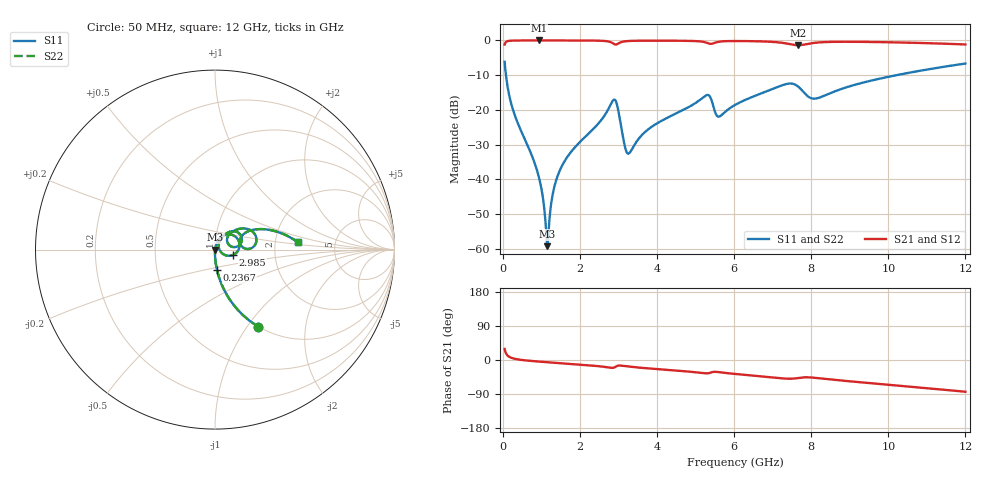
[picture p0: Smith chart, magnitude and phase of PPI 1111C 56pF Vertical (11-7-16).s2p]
# GHz S MA R 50
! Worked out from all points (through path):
!   1601 points, 50 MHz to 12 GHz, reference 50 ohm
!   highest |S21| = -0.01 dB at 938.8 MHz (marker M1); lowest = -1.4 dB at 7.661 GHz (marker M2)
!   group delay of S21, straight-line fit = 19.3 ps
!   lowest |S11| = -59.3 dB at 1.155 GHz (marker M3), VSWR 1.00, Z = 50.1 - j0.0227 ohm
!   |S11| at or under -10 dB: 84.54 MHz to 10.22 GHz (10.13 GHz wide, 197 % of centre)
!   |S22| runs from -59.3 to -6.2 dB; largest |S21 - S12| = 0
!   S11 on the Smith chart (normalised r, x): 50 MHz: 1.00, -1.13; 236.7 MHz: 1.00, -0.23; 2.985 GHz: 1.22, -0.07; 12 GHz: 2.70, +0.28
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0.05  0.492 -60.8  0.8703 29.2  0.8703 29.2  0.492 -60.8
0.2367188  0.114 -84.4  0.9929 5.3  0.9929 5.3  0.114 -84.4
0.9387813  0.01072 -89.0  0.9989 -4.2  0.9989 -4.2  0.01072 -89.0
1.028406  0.006133 -85.4  0.9989 -4.9  0.9989 -4.9  0.006133 -85.4
1.155375  0.001084 -12.1  0.9989 -5.9  0.9989 -5.9  0.001084 -12.1
1.192719  0.00188 48.1  0.9988 -6.2  0.9988 -6.2  0.00188 48.1
1.30475  0.006359 72.4  0.9987 -7.1  0.9987 -7.1  0.006359 72.4
1.439188  0.01172 75.8  0.9986 -8.0  0.9986 -8.0  0.01172 75.8
2.044156  0.03623 74.2  0.9971 -12.5  0.9971 -12.5  0.03623 74.2
2.85825  0.1357 30.9  0.9099 -20.7  0.9099 -20.7  0.1357 30.9
2.985219  0.106 -16.1  0.8938 -15.1  0.8938 -15.1  0.106 -16.1
3.164469  0.03042 -16.2  0.9694 -16.1  0.9694 -16.1  0.03042 -16.2
3.254094  0.02333 15.2  0.98 -17.3  0.98 -17.3  0.02333 15.2
4.038312  0.06545 60.8  0.9919 -24.2  0.9919 -24.2  0.06545 60.8
5.285594  0.1627 32.8  0.9275 -35.2  0.9275 -35.2  0.1627 32.8
5.591812  0.07968 25.4  0.9543 -31.9  0.9543 -31.9  0.07968 25.4
6.025  0.1175 46.9  0.9799 -36.8  0.9799 -36.8  0.1175 46.9
7.302156  0.231 26.1  0.9147 -48.9  0.9147 -48.9  0.231 26.1
7.660656  0.2168 4.6  0.8518 -47.5  0.8518 -47.5  0.2168 4.6
8.019156  0.1461 10.6  0.9124 -46.3  0.9124 -46.3  0.1461 10.6
10.01331  0.3 22.2  0.941 -65.4  0.941 -65.4  0.3 22.2
12  0.4646 4.9  0.8748 -83.8  0.8748 -83.8  0.4646 4.9
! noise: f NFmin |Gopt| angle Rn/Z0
0.05  0.0003756  0.8674  0.5859  0.0006088
1.372  0.003976  0.6895  7  0.002482
2.701  0.02314  0.8839  13.75  0.04262
4.031  0.01462  0.7492  20.26  0.01138
5.36  0.07012  0.925  26.87  0.1959
6.682  0.03075  0.8048  32.92  0.03013
8.012  0.07748  0.9047  39.21  0.1583
9.341  0.0359  0.7828  44.66  0.02909
10.67  0.03209  0.739  49.73  0.02037
12  0.03303  0.728  54.56  0.01921
